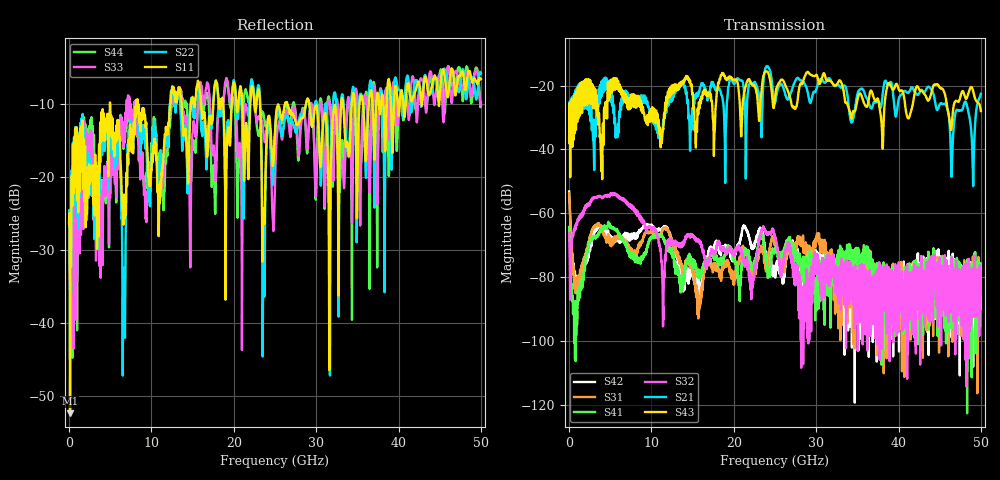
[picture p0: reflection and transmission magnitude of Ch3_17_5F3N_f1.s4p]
!Agilent Technologies,N5247A,US51170199,A.09.90.13
!Agilent N5247A: A.09.90.13
!Date: Wednesday, December 09, 2015 09:44:10
!Correction: S11(Full 4 Port(1,2,3,4))
!S12(Full 4 Port(1,2,3,4))
!S13(Full 4 Port(1,2,3,4))
!S14(Full 4 Port(1,2,3,4))
!S21(Full 4 Port(1,2,3,4))
!S22(Full 4 Port(1,2,3,4))
!S23(Full 4 Port(1,2,3,4))
!S24(Full 4 Port(1,2,3,4))
!S31(Full 4 Port(1,2,3,4))
!S32(Full 4 Port(1,2,3,4))
!S33(Full 4 Port(1,2,3,4))
!S34(Full 4 Port(1,2,3,4))
!S41(Full 4 Port(1,2,3,4))
!S42(Full 4 Port(1,2,3,4))
!S43(Full 4 Port(1,2,3,4))
!S44(Full 4 Port(1,2,3,4))
!S4P File: Measurements: <S11,S12,S13,S14>,
!<S21,S22,S23,S24>,
!<S31,S32,S33,S34>,
!<S41,S42,S43,S44>:
# Hz S  dB  R 50
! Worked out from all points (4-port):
!   3201 points, 10 MHz to 50 GHz, reference 50 ohm
!   strongest paths, dB at 10 MHz, 12.51 GHz, 25 GHz, 37.5 GHz, 50 GHz:
!     S43: -38.0, -21.4, -24.0, -24.1, -28.0
!     S21: -37.2, -22.5, -25.3, -24.8, -22.6
!     S32: -66.1, -69.8, -67.3, -87.0, -82.1
!     S41: -64.2, -72.2, -71.4, -79.6, -89.9
!     S31: -53.6, -69.0, -69.1, -79.2, -78.1
!     S42: -53.1, -68.8, -78.1, -83.3, -80.8
!   lowest |S11| = -52.4 dB at 119.4 MHz (marker M1), VSWR 1.00, Z = 50.1 + j0.232 ohm
!   |S11| at or under -10 dB: start of sweep to 4.961 GHz; 8.347 GHz to 12.32 GHz (3.971 GHz wide, 38.4 % of centre); 29.17 GHz to 33.03 GHz (3.864 GHz wide, 12.4 % of centre)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
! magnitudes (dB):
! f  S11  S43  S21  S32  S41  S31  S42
! 10 MHz  -26.4  -38.0  -37.2  -66.1  -64.2  -53.6  -53.1
! 119.4 MHz  -52.4  -35.0  -36.2  -83.7  -71.8  -59.6  -59.9
! 838 MHz  -19.4  -33.9  -30.8  -64.4  -92.2  -82.7  -84.6
! 6.649 GHz  -24.0  -23.8  -23.2  -55.8  -68.8  -68.0  -66.7
! 8.227 GHz  -11.1  -24.0  -25.8  -59.7  -73.8  -71.9  -66.3
! 23.65 GHz  -24.5  -16.6  -17.4  -64.6  -69.2  -72.8  -68.0
! 50 GHz  -6.6  -28.0  -22.6  -82.1  -89.9  -78.1  -80.8
